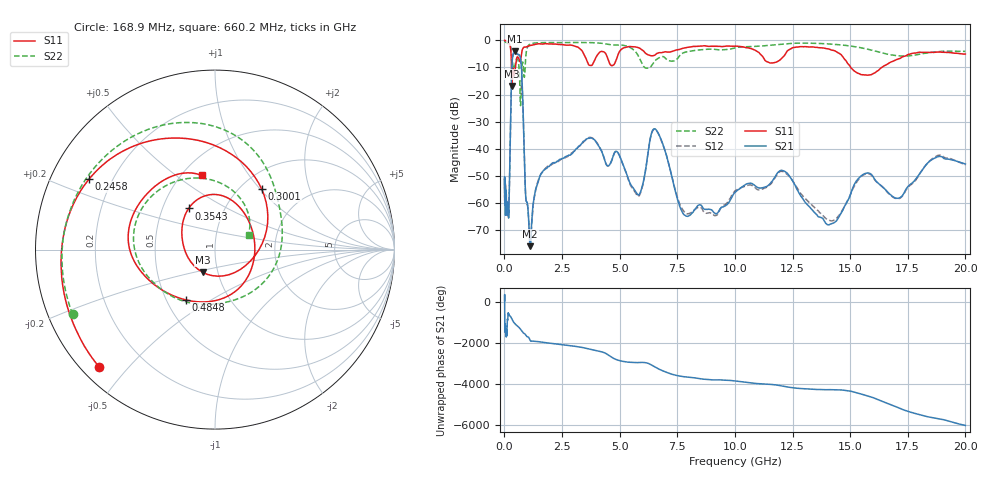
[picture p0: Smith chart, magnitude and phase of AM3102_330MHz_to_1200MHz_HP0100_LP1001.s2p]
! Date/Time: Tue, Sep 11, 2018 5:13 PM
! Network Analyzer: Agilent Technologies E8362B Rev: A.07.50.63
! Sweep from 0.010 to 20.000 GHz, 1601 Points, Sweep Type: LOG
! Power Supply: 4.949 V, 0.001 A
# Hz S DB R 50
!freq MagS11 AngS11 MagS21 AngS21 MagS12 AngS12 MagS22 AngS22
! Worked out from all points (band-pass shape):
!   1601 points, 10 MHz to 20 GHz, reference 50 ohm
!   highest |S21| = -4.02 dB at 449.3 MHz (marker M1); lowest = -76.1 dB at 1.124 GHz (marker M2)
!   |S21| within 3 dB of the highest: 344.3 MHz to 705.3 MHz (361 MHz wide, 68.8 % of centre)
!   lowest |S11| = -16.8 dB at 330 MHz (marker M3), VSWR 1.34, Z = 42.2 - j10.9 ohm
!   |S11| at or under -10 dB: 308 MHz to 481.5 MHz (173.5 MHz wide, 43.9 % of centre); 15.03 GHz to 16.37 GHz (1.345 GHz wide, 8.57 % of centre)
!   |S22| runs from -24.1 to -0.3 dB; largest |S21 - S12| = 0.012
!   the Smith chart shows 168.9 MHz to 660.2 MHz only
!   S11 on the Smith chart (normalised r, x): 168.9 MHz: 0.05, -0.42; 245.8 MHz: 0.12, +0.26; 300.1 MHz: 1.24, +1.02; 354.3 MHz: 0.68, +0.34; 484.8 MHz: 0.62, -0.39; 660.2 MHz: 0.62, +0.62
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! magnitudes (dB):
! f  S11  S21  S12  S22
! 10 MHz  0.0  -51.7  -51.2  -0.3
! 35.55 MHz  0.0  -58.8  -58.5  -0.5
! 126.4 MHz  -0.4  -64.0  -62.7  -1.0
! 168.9 MHz  -0.7  -63.0  -63.6  -1.2
! 245.8 MHz  -1.9  -41.0  -41.0  -1.9
! 300.1 MHz  -7.4  -16.8  -16.9  -3.6
! 330 MHz  -16.8  -8.7  -8.7  -6.5
! 354.3 MHz  -11.3  -6.3  -6.4  -8.3
! 447.2 MHz  -11.9  -4.0  -4.1  -9.6
! 449.3 MHz  -11.8  -4.0  -4.1  -9.5
! 484.8 MHz  -9.8  -4.1  -4.2  -8.3
! 660.2 MHz  -7.5  -5.5  -5.6  -13.8
! 754.2 MHz  -4.3  -12.8  -12.8  -11.2
! 1.124 GHz  -1.9  -76.1  -74.0  -1.3
! 1.59 GHz  -1.3  -49.3  -49.3  -0.8
! 3.757 GHz  -9.3  -36.0  -35.9  -0.8
! 5.652 GHz  -2.4  -55.3  -55.9  -3.9
! 6.549 GHz  -5.3  -32.8  -32.9  -7.4
! 7.92 GHz  -2.6  -65.0  -64.1  -4.2
! 12.03 GHz  -6.6  -48.0  -48.4  -1.4
! 14.07 GHz  -3.2  -68.2  -66.4  -1.3
! 20 GHz  -5.0  -45.7  -46.1  -4.0
